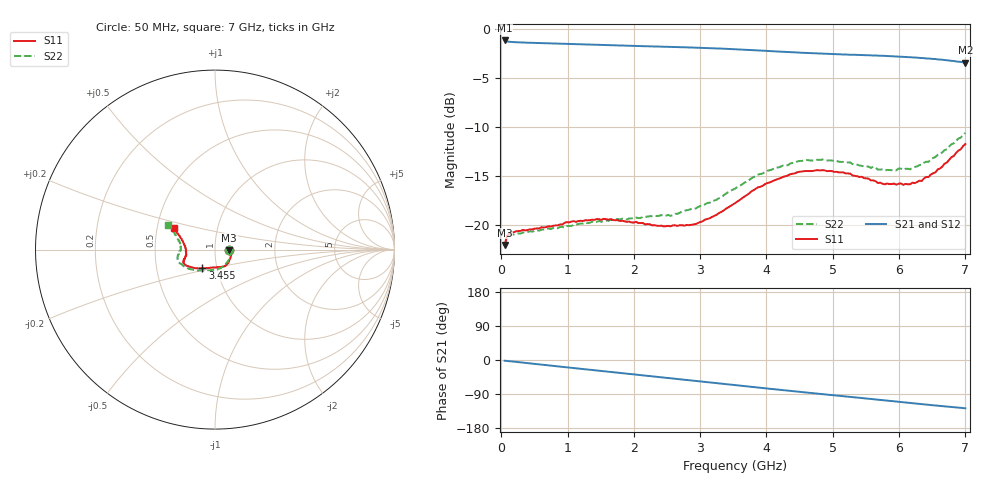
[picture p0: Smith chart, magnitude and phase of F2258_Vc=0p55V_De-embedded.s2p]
! Integrated Device Technology
! Corporate Headquarters
! 6024 Silver Creek Valley Road
! San Jose, CA 95138  USA
! Phone:  1-408-284-8200
! Toll Free:  1-800-223-1366
! Webpage:  http://www.idt.com/
! Timing and RF Division
! 515 Groton Road, Suite 102
! Westford, MA 01886-6024
! Device:  F2258
! Description: Voltage Variable RF Attenuator
! Frequency:  50.0 -  6000.00 MHz
! Package:  3x3 mm Thin QFN Plastic Package: 16 pin
! Ports:  2 RF, 2 DC
!  Pin  1  = NC
!  Pin  2  = NC
!  Pin  3  = RF2  = Port 2
!  Pin  4  = GND
!  Pin  5  = Vdd
!  Pin  6  = NC
!  Pin  7  = VCTRL
!  Pin  8  = NC
!  Pin  9  = GND
!  Pin 10  = RF1  = Port 1
!  Pin 11  = NC
!  Pin 12  = NC
!  Pin 13  = NC
!  Pin 14  = NC
!  Pin 15  = NC
!  Pin 16  = NC
! Vcntrl:  0.550 Volts
! Vdd:  +3.300 Volts
! Current:  1.103 mA
! Data:  The device was measured on a the F2258 evaluation board which has
!  individual transmission lines to the RF pins.  Data was collected
!  using a calibrated network analyzer.  The evaluation board was
!  de-embedded using a TRL calibration technique.
!  The reference plane is the edge of the package pin.
! Misc:  SN 10
!  Action Tracker AT0285
! Date Measured:  2014-12-10
! Date:  2016-01-13  MJV
! Note:
!  Integrated Device Technology supplies this data as a sample of measured
!  data at the package pin for this product.  Your particular data for this
!  product may vary.
!  Data was taken at 25 degrees C.
!  Integrated Device Technology reserves the right to change this data at anytime.
!Freq_(GHz)  S11M_(dB)  S11P_(deg)  S21M_(dB)  S21P_(deg)  S12M_(dB)  S12P_(deg)  S22M_(dB)  S22P_(deg)
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# GHz S dB R 50
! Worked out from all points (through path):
!   201 points, 50 MHz to 7 GHz, reference 50 ohm
!   highest |S21| = -1.17 dB at 50 MHz (marker M1); lowest = -3.4 dB at 7 GHz (marker M2)
!   group delay of S21, straight-line fit = 50.5 ps
!   lowest |S11| = -22.0 dB at 50 MHz (marker M3), VSWR 1.17, Z = 58.6 - j0.48 ohm
!   |S11| at or under -10 dB: start of sweep to end of sweep
!   |S22| runs from -22.1 to -10.6 dB; largest |S21 - S12| = 0.0004
!   S11 on the Smith chart (normalised r, x): 50 MHz: 1.17, -0.01; 3.455 GHz: 0.85, -0.18; 7 GHz: 0.61, +0.16
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0.05  -22.02 -2.9  -1.17 -2.0  -1.17 -2.0  -22.15 -2.9
0.08475  -21.13 -4.7  -1.26 -2.5  -1.27 -2.5  -21.28 -4.7
0.15425  -20.71 -7.2  -1.33 -3.7  -1.33 -3.7  -20.95 -8.2
0.71025  -20.12 -30.2  -1.46 -14.1  -1.46 -14.1  -20.35 -34.1
1.2315  -19.58 -49.5  -1.57 -23.9  -1.57 -23.9  -19.84 -57.3
1.6485  -19.38 -60.1  -1.66 -31.5  -1.66 -31.5  -19.48 -70.4
2.37825  -20.09 -78.7  -1.79 -44.8  -1.79 -44.8  -19.06 -89.2
2.552  -20.12 -84.2  -1.83 -48.0  -1.82 -48.0  -19.06 -94.5
2.93425  -19.89 -100.5  -1.90 -55.1  -1.90 -55.1  -18.30 -108.1
3.247  -18.95 -114.3  -1.98 -61.0  -1.98 -61.0  -17.42 -120.6
3.4555  -18.06 -124.1  -2.04 -64.9  -2.04 -64.9  -16.51 -128.4
3.525  -17.77 -126.6  -2.06 -66.2  -2.06 -66.2  -16.28 -131.5
4.0115  -15.72 -142.7  -2.24 -75.3  -2.24 -75.3  -14.46 -147.7
4.46325  -14.61 -152.3  -2.40 -83.4  -2.40 -83.4  -13.51 -159.3
4.7065  -14.47 -155.7  -2.47 -87.7  -2.48 -87.7  -13.41 -163.7
5.2625  -14.74 -162.2  -2.63 -97.4  -2.63 -97.4  -13.61 -172.2
5.6795  -15.71 -168.0  -2.72 -104.6  -2.71 -104.6  -14.34 -177.9
5.85325  -15.82 -172.3  -2.77 -107.7  -2.77 -107.7  -14.38 177.4
6.166  -15.84 179.6  -2.88 -113.3  -2.88 -113.3  -14.31 171.2
6.33975  -15.50 172.7  -2.96 -116.4  -2.96 -116.4  -13.83 166.7
6.6525  -14.03 161.8  -3.13 -121.9  -3.14 -121.9  -12.58 159.8
7  -11.73 152.5  -3.43 -127.4  -3.44 -127.4  -10.59 152.3
